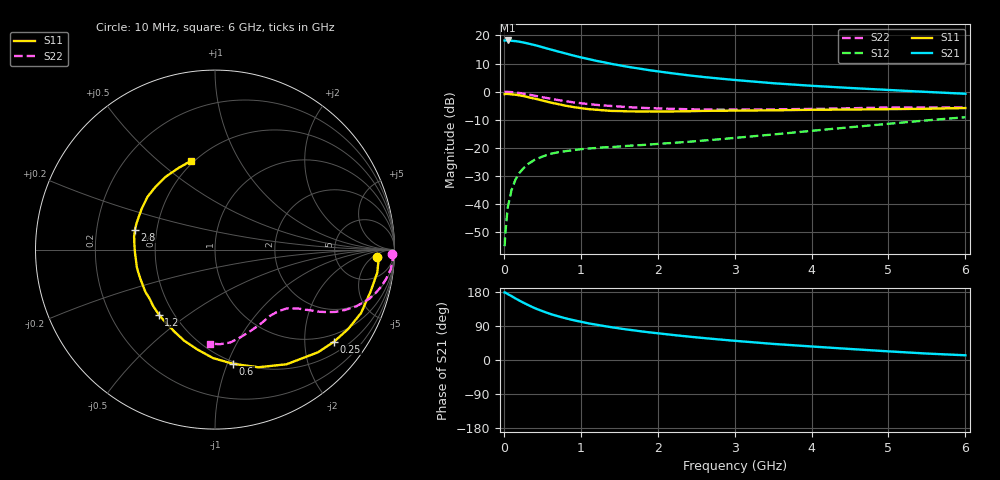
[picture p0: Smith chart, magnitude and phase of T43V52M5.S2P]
! Infineon Technologies  Discrete & RF Semiconductors
! BFR182T
! Si NPN RF Bipolar Junction Transistor in SC75
! VCE = 3.5 V  IC = 2.5 mA
! Common Emitter S-Parameters:  October  1999
# GHz  S  MA  R  50
!  f  S11  S21  S12  S22
! GHz  MAG  ANG  MAG  ANG  MAG  ANG  MAG  ANG
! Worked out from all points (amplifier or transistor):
!   36 points, 10 MHz to 6 GHz, reference 50 ohm
!   highest |S21| = 18.2 dB at 50 MHz (marker M1)
!   |S21| within 3 dB of that: start of sweep to 581.6 MHz
!   unconditionally stable (mu >= 1): 1.852 GHz to 4.259 GHz
!   at 250 MHz: K = 0.17, MSG = 22.4 dB, |S12| = -27.4 dB
!   at 1.4 GHz: K = 0.84, MSG = 14.8 dB, |S12| = -19.7 dB
!   at 6 GHz: K = 0.83, MSG = 4.2 dB, |S12| = -9.1 dB
!   lowest NFmin = 1.10 dB at 450 MHz
!   S11 on the Smith chart (normalised r, x): 10 MHz: 16, -7; 250 MHz: 0.79, -2.73; 600 MHz: 0.48, -1.05; 1.2 GHz: 0.42, -0.39; 2.8 GHz: 0.38, +0.11; 6 GHz: 0.48, +0.65
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0.01  0.9037 -2.6  8.132 178.2  0.0018 75.9  0.9891 -1.4
0.02  0.9145 -1.9  8.14 177.9  0.0031 99.2  0.9974 -1.4
0.05  0.9131 -8.1  8.15 174.1  0.0087 89.4  0.9917 -3.3
0.1  0.8975 -15.3  8.039 168.6  0.0179 82.5  0.9845 -6.5
0.15  0.8871 -23.5  7.93 162.6  0.0272 76.8  0.9673 -9.7
0.25  0.8386 -37.7  7.521 151.7  0.0428 69.7  0.9262 -15.2
0.3  0.8104 -44.9  7.267 146.6  0.0504 66.7  0.9029 -17.6
0.4  0.7532 -58.0  6.751 137.0  0.0617 60.8  0.8498 -21.8
0.5  0.6988 -69.7  6.194 129.1  0.0702 55.8  0.8008 -24.8
0.6  0.6448 -80.9  5.678 121.8  0.0784 52.0  0.7547 -27.4
0.7  0.6047 -91.0  5.208 115.7  0.0838 49.5  0.7134 -29.2
0.8  0.5654 -99.9  4.797 110.2  0.0877 47.3  0.6789 -30.7
0.9  0.5355 -108.8  4.414 105.3  0.0915 45.8  0.6483 -31.8
1.1  0.4912 -124.0  3.808 96.7  0.0979 44.3  0.6032 -33.7
1.2  0.4787 -130.8  3.547 93.3  0.1 43.8  0.5846 -34.5
1.6  0.4483 -154.3  2.79 80.5  0.109 44.5  0.5343 -37.6
2.2  0.4462 -177.6  2.117 66.0  0.1233 48.7  0.4965 -43.4
2.8  0.4595 166.0  1.715 54.2  0.1427 53.3  0.4798 -50.5
3.5  0.4675 151.1  1.417 42.5  0.1737 57.3  0.4865 -59.5
4.5  0.4819 133.6  1.166 29.1  0.2338 58.9  0.5083 -73.6
5.5  0.4979 114.2  0.992 17.0  0.3098 56.2  0.5279 -87.1
6  0.5129 104.8  0.92 12.4  0.3522 53.2  0.5241 -93.1
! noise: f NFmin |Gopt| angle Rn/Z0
0.45  1.1  0.39  29  0.35
0.9  1.2  0.37  59  0.28
1.8  1.8  0.28  128  0.2
